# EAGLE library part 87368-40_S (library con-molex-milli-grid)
RECEPTACAL
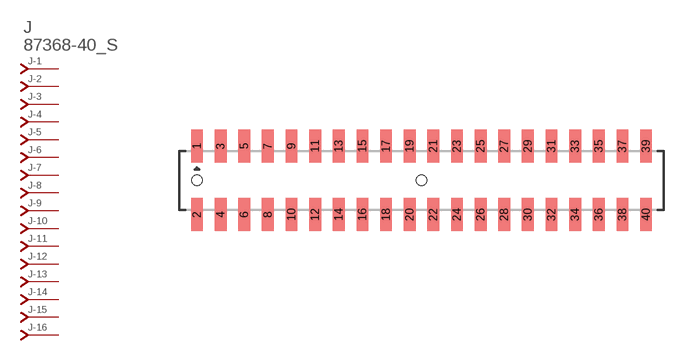
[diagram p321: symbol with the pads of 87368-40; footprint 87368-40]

Designator prefix J; gates -1=J-NV -2=J-N -3=J-N -4=J-N -5=J-N -6=J-N -7=J-N -8=J-N -9=J-N -10=J-N -11=J-N -12=J-N -13=J-N -14=J-N -15=J-N -16=J-N -17=J-N -18=J-N -19=J-N -20=J-N -21=J-N -22=J-N -23=J-N -24=J-N -25=J-N -26=J-N -27=J-N -28=J-N -29=J-N -30=J-N -31=J-N -32=J-N -33=J-N -34=J-N -35=J-N -36=J-N -37=J-N -38=J-N -39=J-N -40=J-N

## 87368-40_S  [87368-40]
1  -1:J  pas
2  -2:J  pas
3  -3:J  pas
4  -4:J  pas
5  -5:J  pas
6  -6:J  pas
7  -7:J  pas
8  -8:J  pas
9  -9:J  pas
10  -10:J  pas
11  -11:J  pas
12  -12:J  pas
13  -13:J  pas
14  -14:J  pas
15  -15:J  pas
16  -16:J  pas
17  -17:J  pas
18  -18:J  pas
19  -19:J  pas
20  -20:J  pas
21  -21:J  pas
22  -22:J  pas
23  -23:J  pas
24  -24:J  pas
25  -25:J  pas
26  -26:J  pas
27  -27:J  pas
28  -28:J  pas
29  -29:J  pas
30  -30:J  pas
31  -31:J  pas
32  -32:J  pas
33  -33:J  pas
34  -34:J  pas
35  -35:J  pas
36  -36:J  pas
37  -37:J  pas
38  -38:J  pas
39  -39:J  pas
40  -40:J  pas

## Footprint 87368-40 (pad centres in mm)
RECEPTACAL SMD Dual Row, Side Entry
smd 1 x 2.8: 1 -19,2.9; 2 -19,-2.9; 3 -17,2.9; 4 -17,-2.9; 5 -15,2.9; 6 -15,-2.9; 7 -13,2.9; 8 -13,-2.9; 9 -11,2.9; 10 -11,-2.9; 11 -9,2.9; 12 -9,-2.9; 13 -7,2.9; 14 -7,-2.9; 15 -5,2.9; 16 -5,-2.9; 17 -3,2.9; 18 -3,-2.9; 19 -1,2.9; 20 -1,-2.9; 21 1,2.9; 22 1,-2.9; 23 3,2.9; 24 3,-2.9; 25 5,2.9; 26 5,-2.9; 27 7,2.9; 28 7,-2.9; 29 9,2.9; 30 9,-2.9; 31 11,2.9; 32 11,-2.9; 33 13,2.9; 34 13,-2.9; 35 15,2.9; 36 15,-2.9; 37 17,2.9; 38 17,-2.9; 39 19,2.9; 40 19,-2.9
hole 0.914 at -19,0
hole 0.914 at 0,0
